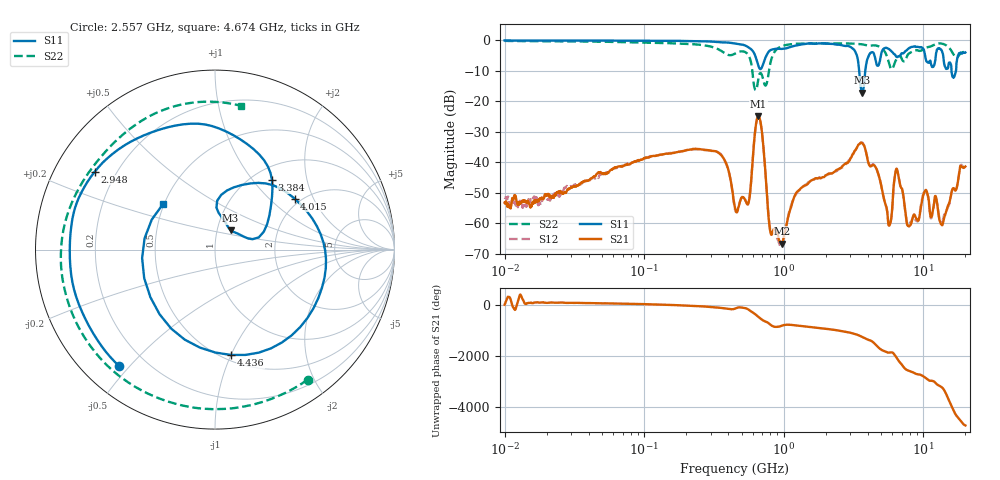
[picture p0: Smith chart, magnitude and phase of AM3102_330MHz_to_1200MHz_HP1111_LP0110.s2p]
! Date/Time: Tue, Sep 11, 2018 5:24 PM
! Network Analyzer: Agilent Technologies E8362B Rev: A.07.50.63
! Sweep from 0.010 to 20.000 GHz, 1601 Points, Sweep Type: LOG
! Power Supply: 4.949 V, 0.001 A
# Hz S DB R 50
!freq MagS11 AngS11 MagS21 AngS21 MagS12 AngS12 MagS22 AngS22
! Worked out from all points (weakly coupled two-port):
!   1601 points, 10 MHz to 20 GHz, reference 50 ohm
!   highest |S21| = -24.90 dB at 657.1 MHz (marker M1); lowest = -66.6 dB at 970.1 MHz (marker M2)
!   lowest |S11| = -17.2 dB at 3.651 GHz (marker M3), VSWR 1.32, Z = 58 + j12.8 ohm
!   |S11| at or under -10 dB: 3.468 GHz to 3.835 GHz (366.3 MHz wide, 10 % of centre); 15.91 GHz to 17.11 GHz (1.206 GHz wide, 7.31 % of centre)
!   |S22| runs from -16.3 to -0.2 dB; largest |S21 - S12| = 0.005
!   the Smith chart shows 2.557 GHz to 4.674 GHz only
!   S11 on the Smith chart (normalised r, x): 2.557 GHz: 0.11, -0.47; 2.948 GHz: 0.12, +0.29; 3.384 GHz: 1.22, +1.26; 4.015 GHz: 1.85, +1.45; 4.436 GHz: 0.55, -1.00; 4.674 GHz: 0.49, +0.30
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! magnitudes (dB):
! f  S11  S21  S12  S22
! 10 MHz  0.0  -53.2  -51.6  -0.2
! 35.55 MHz  -0.1  -46.7  -47.0  -0.4
! 126.4 MHz  -0.2  -37.7  -37.7  -0.8
! 342.8 MHz  -0.6  -37.0  -36.8  -3.0
! 447.2 MHz  -1.0  -54.9  -55.5  -4.3
! 559.1 MHz  -2.3  -53.3  -53.2  -4.9
! 657.1 MHz  -8.3  -24.9  -24.9  -12.4
! 798.4 MHz  -3.3  -62.5  -61.9  -7.8
! 970.1 MHz  -2.8  -66.6  -66.6  -1.9
! 1.59 GHz  -1.1  -45.9  -45.8  -1.0
! 2.557 GHz  -1.5  -41.9  -41.9  -1.0
! 2.948 GHz  -2.0  -39.6  -39.3  -1.0
! 3.384 GHz  -6.0  -34.6  -34.8  -1.2
! 3.651 GHz  -17.2  -33.7  -33.5  -1.3
! 4.015 GHz  -5.6  -39.8  -39.6  -1.7
! 4.436 GHz  -4.5  -41.0  -40.8  -1.6
! 4.674 GHz  -8.3  -42.8  -42.9  -1.8
! 5.652 GHz  -2.8  -60.7  -60.7  -7.2
! 6.426 GHz  -5.4  -42.0  -42.4  -6.1
! 7.845 GHz  -2.7  -60.9  -60.1  -4.4
! 13.48 GHz  -3.3  -60.4  -59.2  -1.0
! 20 GHz  -4.0  -41.4  -41.9  -3.8
